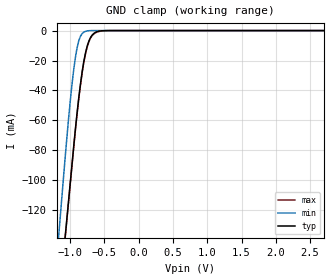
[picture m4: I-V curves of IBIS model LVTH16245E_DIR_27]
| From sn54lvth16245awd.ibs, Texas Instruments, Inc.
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[Model]   LVTH16245E_DIR_27
Model_type  Input
Vinl = 0.8
Vinh = 2
| variable   typ   min   max
C_comp   3.73pF   2.62pF   4.57pF
[Temperature Range]   40   -40   100
| Ambient temperature   25   -40   85
[Voltage range]   2.7   2.7   2.7
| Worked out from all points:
|   GND clamp passes 1 mA (typ) near -0.62 V on its own axis
[GND Clamp]
| LVTH16245E_DIR_27
|   Voltage   I(typ)   I(min)   I(max)
-5V       -2.043A    -2.266A    -2.044A
-1.175V   -186.8mA   -140.7mA   -187.5mA
-1.155V   -177.1mA   -129.6mA   -177.8mA
-1.075V   -138.3mA   -85.25mA   -139.1mA
-1.05V    -126.2mA   -72.09mA   -126.9mA
-975mV    -89.84mA   -36.15mA   -90.57mA
-900mV    -55.04mA   -11.48mA   -55.73mA
-825mV    -27.27mA   -1.973mA   -27.9mA
-775mV    -14.55mA   -465.3uA   -15.13mA
-725mV    -6.68mA    -70.56uA   -7.152mA
-650mV    -1.713mA   -2.477uA   -2.065mA
2.7V      13.81pA    2.798pA    2.893nA
